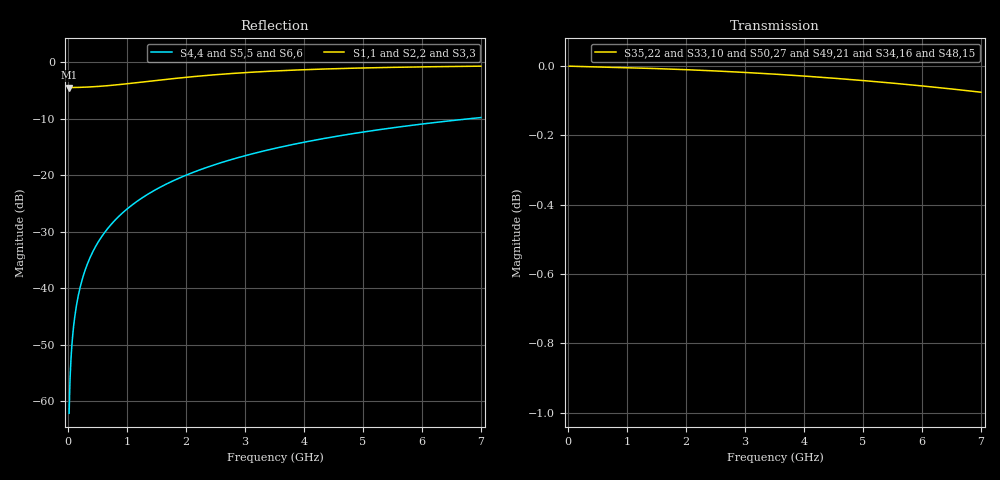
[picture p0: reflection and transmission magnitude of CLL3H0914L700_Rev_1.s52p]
! Touchstone file exported from HFSS 2018.2.0
!  File:  /home/rfpwrbs_nlv03685/HFSS/CLL3H0914L700_Rev_0/CLL3H0914L700_Rev_1.aedt
!  Generated:  9:01:19 AM  Jul 22, 2020
!  Design:  04a_SOT502B2
!  Project:  CLL3H0914L700_Rev_1
!  Setup:  Setup1
!  Solution:  Sweep
! Variables:
!  AirBox_H = 45mm
!  AirBox_L = 40mm
!  AirBox_W = 140mm
!  BW_Dia = 50um
!  Back_Metal_H = 0.03mm
!  CpoMetalYOffset = 0.182mm
!  CpoMetal_L = 0.4mm
!  CpoMetal_W = 4.6mm
!  CpoOxide_H = 0.64um
!  CpoYOffset = 0.919mm
!  Cpo_H = 50um
!  Cpo_L = 0.765mm
!  CprMetalYOffset = 0.283mm
!  CprMetal_L = 0.18mm
!  CprMetal_W = 4.8mm
!  CprOxide_H = 2um
!  CprYOffset = 1.051mm
!  Cpr_H = 200um
!  Cpr_L = 0.765mm
!  DIEDrMetalYOffset = 1176um
!  DIEDrMetal_L = 0.16mm
!  DIEDrMetal_W = 4.6mm
!  DIEGtMetalYOffset = 0.11mm
!  DIEGtMetal_L = 0.16mm
!  DIEGtMetal_W = 4.6mm
!  DIEMetal_H = 3um
!  DIEOxide_H = 10um
!  DIE_H = 50um
!  DIE_L = 1.45mm
!  DIE_W = 4.9mm
!  DIE_X_Pos = -7.6mm
!  DIE_X_Sep = 5.4mm
!  DIE_Y_Pos = -0.485mm
!  IntPortSep = 150um
!  IntPort_W = 800um
!  Ld_H = 150um
!  Ld_Len = 2.579mm
!  Ld_Sp1 = 167um
!  Ld_Sp2 = 1840um
!  Ld_X_Offset1 = 214um
!  Ld_X_Offset2 = 1043um
!  Lg1_H = 720um
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# GHZ S MA R 50.000000
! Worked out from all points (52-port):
!   450 points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, 15.56 MHz to 7 GHz, reference per port
!   strongest paths, dB at 15.56 MHz, 1.758 GHz, 3.516 GHz, 5.258 GHz, 7 GHz:
!     S35,22: 0.0, 0.0, 0.0, 0.0, -0.1
!     S33,10: 0.0, 0.0, 0.0, 0.0, -0.1
!     S50,27: 0.0, 0.0, 0.0, 0.0, -0.1
!     S49,21: 0.0, 0.0, 0.0, 0.0, -0.1
!     S34,16: 0.0, 0.0, 0.0, 0.0, -0.1
!     S48,15: 0.0, 0.0, 0.0, 0.0, -0.1
!   lowest |S11| = -4.4 dB at 15.56 MHz (marker M1), VSWR 4.00
!   |S11| at or under -10 dB: nowhere
